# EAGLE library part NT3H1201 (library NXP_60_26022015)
NTAG I²C, NFC Forum type 2 Tag compliant IC with I²C interface The NTAG I2C is the first product of NXP’s NTAG family offering both contactless and contact interfaces (see Figure 1). In addition to the passive NFC Forum compliant contactless interface, the IC features an I²C contact interface, which can communicate with a microcontroller if the NTAG I2C is powered from an external power supply. An additional externally powered SRAM mapped into the memory allows a fast data transfer between the RF and I²C interfaces and vice versa, without the write cycle limitations of the EEPROM memory. The NTAG I2C product features a configurable Field Detection Pin, which provides a trigger to an external device depending on the activities at the RF interface. The NTAG I2C product can also supply power to external (low power) devices (e.g., a microcontroller) via the embedded energy harvesting circuitry AAL Eindhoven MK
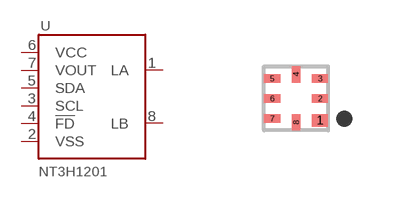
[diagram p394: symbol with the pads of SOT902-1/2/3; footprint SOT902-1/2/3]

Designator prefix U

## NT3H1201W0FHK  [SOT902-1/2/3]
1  LA
2  VSS
3  SCL
4  !FD
5  SDA
6  VCC
7  VOUT
8  LB

## Footprint SOT902-1/2/3 (pad centres in mm)
SOT902-1/2/3 XQFN8U: plastic extremely thin quad flat package; no leads; 8 terminals; UTLP based; body 1.6 x 1.6 x 0.5 mm JEDEC: -- IEC: ---
smd 0.4 x 0.32: 1 0.6,-0.55
smd 0.4 x 0.22: 2 0.6,0; 3 0.6,0.5; 5 -0.6,0.5; 6 -0.6,0; 7 -0.6,-0.5
smd 0.22 x 0.4: 4 0,0.6; 8 0,-0.6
